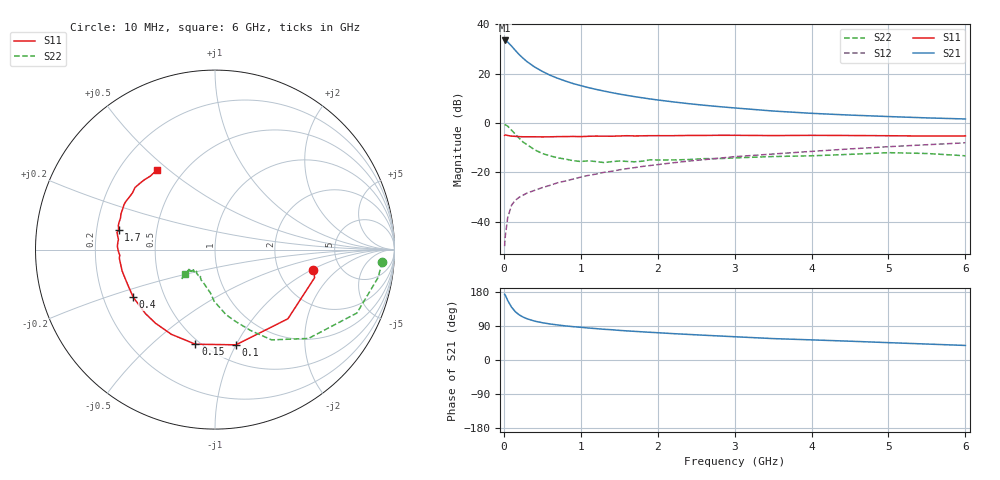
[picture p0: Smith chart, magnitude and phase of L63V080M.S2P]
!  INFINEON TECHNOLOGIES Small Signal Semiconductors
! BFR380L3 , Si-NPN RF-Transistor in TSLP-3-1
!  Vce=3 V,  Ic=80 mA
! Common Emitter S-Parameters:  07. March 2005
#  GHz  S  MA  R  50
! f  S11  S21  S12  S22
! GHz  Mag  Ang  Mag  Ang  Mag  Ang  Mag  Ang
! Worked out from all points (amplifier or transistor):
!   36 points, 10 MHz to 6 GHz, reference 50 ohm
!   highest |S21| = 33.5 dB at 10 MHz (marker M1)
!   |S21| within 3 dB of that: start of sweep to 120.5 MHz
!   unconditionally stable (mu >= 1): 1.159 GHz to 4.873 GHz
!   at 250 MHz: K = 0.56, MSG = 27.7 dB, |S12| = -29.2 dB
!   at 1.4 GHz: K = 1.02, MAG = 15.0 dB, |S12| = -19.5 dB
!   at 6 GHz: K = 0.97, MSG = 4.8 dB, |S12| = -8.0 dB
!   S11 on the Smith chart (normalised r, x): 10 MHz: 3.16, -1.06; 100 MHz: 0.66, -1.00; 150 MHz: 0.47, -0.70; 400 MHz: 0.33, -0.24; 1.7 GHz: 0.29, +0.09; 6 GHz: 0.36, +0.45
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0.01  0.5606 -11.8  47.21 173.6  0.0032 74.4  0.9336 -4.2
0.02  0.5767 -15.7  46.52 170.8  0.0053 83.9  0.9222 -9.7
0.05  0.56 -43.5  43.76 157.1  0.012 72.4  0.8659 -24.1
0.1  0.5432 -77.6  36.37 139.5  0.0217 62.2  0.7188 -43.5
0.15  0.5383 -101.7  29.59 127.3  0.0273 56.2  0.5938 -57.9
0.2  0.5309 -117.3  24.38 119.1  0.0314 55.0  0.4929 -66.2
0.25  0.5274 -129.0  20.59 113.3  0.0346 52.9  0.4118 -74.6
0.3  0.5265 -137.3  17.62 108.9  0.038 53.8  0.3668 -80.5
0.4  0.5272 -149.7  13.69 102.6  0.0433 55.4  0.2877 -90.9
0.5  0.524 -157.5  11.15 98.4  0.0492 58.7  0.2416 -96.2
0.6  0.5265 -163.1  9.33 95.1  0.0547 60.5  0.2168 -102.3
0.7  0.531 -167.1  8.078 92.4  0.0617 61.8  0.1975 -108.5
0.9  0.5353 -175.0  6.321 88.0  0.0733 64.9  0.1731 -118.4
1.1  0.5396 -179.4  5.227 84.4  0.087 66.3  0.1718 -123.0
1.4  0.5409 174.1  4.144 79.9  0.1054 67.2  0.1651 -129.1
1.7  0.5481 168.6  3.433 75.6  0.125 67.9  0.1643 -136.8
2.2  0.5551 161.5  2.688 69.6  0.1567 67.9  0.1789 -137.2
2.8  0.5654 153.6  2.151 63.4  0.1943 67.4  0.1903 -142.4
3.5  0.5577 145.6  1.754 56.5  0.236 65.1  0.2097 -140.2
4.5  0.5594 139.4  1.451 49.6  0.2994 63.1  0.2323 -139.3
5.5  0.5454 131.3  1.273 42.1  0.364 59.2  0.2417 -138.9
6  0.5487 126.4  1.21 38.4  0.3977 56.8  0.2171 -141.2
